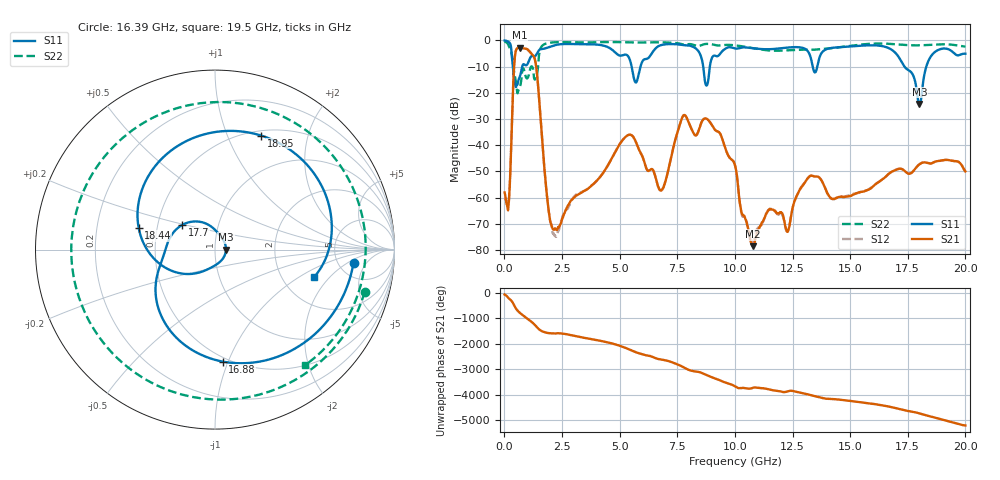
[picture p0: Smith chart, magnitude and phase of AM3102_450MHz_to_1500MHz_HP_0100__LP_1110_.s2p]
!Agilent Technologies,E8364B,MY43040894,A.07.50.67
!Agilent E8364B: A.07.50.67
!Date: Thursday, January 11, 2018 05:38:45
!Correction: S11(Full 2 Port(1,2))
!S21(Full 2 Port(1,2))
!S12(Full 2 Port(1,2))
!S22(Full 2 Port(1,2))
!S2P File: Measurements: S11, S21, S12, S22:
# Hz S  dB  R 50
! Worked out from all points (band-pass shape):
!   1601 points, 10 MHz to 20 GHz, reference 50 ohm
!   highest |S21| = -2.77 dB at 659.7 MHz (marker M1); lowest = -78.5 dB at 10.78 GHz (marker M2)
!   |S21| within 3 dB of the highest: 461.8 MHz to 1.246 GHz (783.9 MHz wide, 91.8 % of centre)
!   lowest |S11| = -24.3 dB at 18 GHz (marker M3), VSWR 1.13, Z = 56.5 + j0.0462 ohm
!   |S11| at or under -10 dB: 367.2 MHz to 774.6 MHz (407.4 MHz wide, 71.4 % of centre); 5.521 GHz to 5.905 GHz (384.4 MHz wide, 6.73 % of centre); 17.36 GHz to 18.31 GHz (949.1 MHz wide, 5.32 % of centre)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
!   |S22| runs from -20.2 to -0.5 dB; largest |S21 - S12| = 0.0027
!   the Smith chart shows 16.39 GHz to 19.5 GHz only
!   S11 on the Smith chart (normalised r, x): 16.39 GHz: 6.97, -2.54; 16.88 GHz: 0.47, -0.96; 17.7 GHz: 0.67, +0.19; 18.44 GHz: 0.39, +0.12; 18.95 GHz: 0.56, +1.33; 19.5 GHz: 3.00, -1.37
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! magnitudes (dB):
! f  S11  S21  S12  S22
! 10 MHz  -0.1  -58.0  -60.0  -0.5
! 184.9 MHz  -0.6  -62.6  -61.5  -2.0
! 447.3 MHz  -15.8  -7.0  -7.0  -13.2
! 659.7 MHz  -14.1  -2.8  -2.8  -18.0
! 1.347 GHz  -5.9  -8.2  -8.2  -14.7
! 2.146 GHz  -2.0  -72.3  -74.0  -0.8
! 3.346 GHz  -1.5  -58.1  -57.9  -0.8
! 5.42 GHz  -6.9  -36.0  -36.0  -0.8
! 6.682 GHz  -2.3  -56.0  -56.1  -0.8
! 7.794 GHz  -1.8  -28.5  -28.5  -1.6
! 10.01 GHz  -3.1  -47.6  -47.7  -1.9
! 10.78 GHz  -3.0  -78.5  -76.8  -3.0
! 13.34 GHz  -8.5  -51.7  -51.6  -3.6
! 16.39 GHz  -2.2  -53.1  -53.2  -1.2
! 16.68 GHz  -3.0  -50.9  -50.9  -1.3
! 16.88 GHz  -4.1  -49.8  -49.8  -1.5
! 17.7 GHz  -12.8  -50.3  -50.2  -1.9
! 18 GHz  -24.3  -47.3  -47.3  -1.9
! 18.44 GHz  -7.1  -47.0  -47.0  -1.7
! 18.95 GHz  -3.3  -45.8  -45.9  -1.5
! 19.5 GHz  -4.8  -46.1  -46.1  -1.8
! 20 GHz  -5.1  -50.0  -50.2  -2.4
